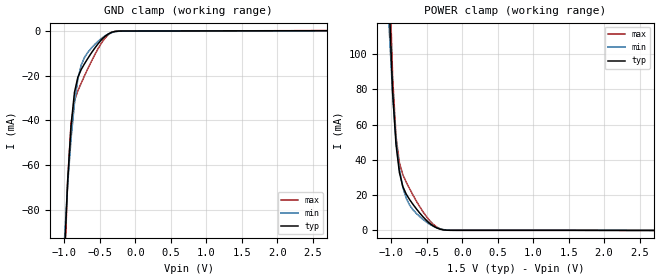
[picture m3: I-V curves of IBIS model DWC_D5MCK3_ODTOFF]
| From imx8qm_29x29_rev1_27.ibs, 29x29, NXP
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[Model] DWC_D5MCK3_ODTOFF
Model_type   Input
Polarity   Non-Inverting
Enable   Active-High
C_comp   1.260pF   1.180pF   1.362pF
C_comp_power_clamp   275.501fF   256.643fF   303.068fF
C_comp_gnd_clamp 982.421fF   918.243fF   1.058pF
Vinh = 875.000mV
Vinl = 625.000mV
[Model Spec]
D_overshoot_ampl_h 0.4 NA   NA
D_overshoot_ampl_l 0.4 NA   NA
D_overshoot_area_l 100.000p NA   NA
D_overshoot_area_h 100.000p NA   NA
[Receiver Thresholds]
Vcross_low = 575.000mV
Vcross_high = 925.000mV
Vdiff_ac = 250.000mV
Vdiff_dc = 200.000mV
Tdiffslew_ac = 10.000ns
[Temperature Range]   25.000   125.000   -40.000
[Voltage Range]   1.500V   1.425V   1.575V
[GND Clamp Reference]   0.00V   0.00V   0.00V
[C Comp Corner]
| variable   typ   min   max
C_comp 1.260pF   1.362pF   1.180pF
C_comp_pullup 275.501fF   303.068fF   256.643fF
C_comp_pulldown 982.421fF   1.058pF   918.243fF
[POWER Clamp Reference]   1.500V   1.425V   1.575V
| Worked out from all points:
|   GND clamp passes 1 mA (typ) near -0.36 V on its own axis
|   POWER clamp passes 1 mA (typ) near -0.34 V on its own axis
[GND Clamp]
-1.48V    -918.2mA   -652.1mA   -1.176A
-1.002V   -101.7mA   -94.77mA   -109.1mA
-954.5mV  -67.02mA   -68.69mA   -66.81mA
-906.8mV  -42.34mA   -48.1mA    -41.42mA
-859.1mV  -27.51mA   -32.38mA   -31.19mA
-811.4mV  -20.68mA   -21.56mA   -26.8mA
-763.6mV  -17.22mA   -15.21mA   -23.29mA
-715.9mV  -14.57mA   -11.71mA   -19.94mA
-429.5mV  -2.409mA   -2.204mA   -3.222mA
-334.1mV  -538.8uA   -707.4uA   -589.3uA
-238.6mV  -34.43uA   -108.5uA   -17.28uA
2.959V    171.1uA    140uA      213.2uA
[Power Clamp]
-1.459V   1.027A     711.2mA    1.35A
-1.03V    129.3mA    114.5mA    151.4mA
-981.8mV  78.48mA    77.22mA    87.29mA
-934.1mV  48.73mA    51.4mA     53.47mA
-886.4mV  32.89mA    34.83mA    38.4mA
-838.6mV  24.91mA    24.53mA    31.7mA
-790.9mV  20.61mA    18.26mA    27.45mA
-743.2mV  17.51mA    14.37mA    23.68mA
-456.8mV  3.892mA    3.387mA    5.399mA
-361.4mV  1.383mA    1.455mA    1.887mA
-218.2mV  56.59uA    161.1uA    60.54uA
2.979V    -85.62uA   -74.93uA   -101.2uA
